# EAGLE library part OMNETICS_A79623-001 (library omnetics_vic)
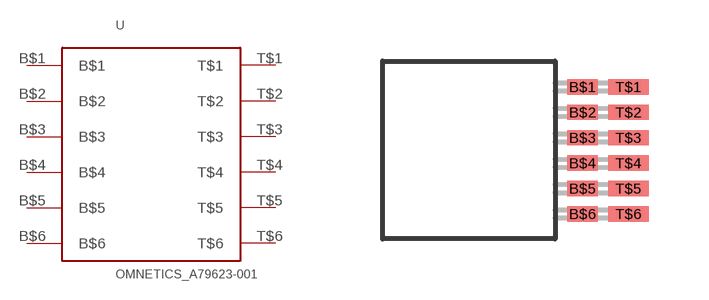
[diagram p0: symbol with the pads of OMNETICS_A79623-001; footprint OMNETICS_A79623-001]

Designator prefix -

## OMNETICS_A79623-001  [OMNETICS_A79623-001]
B$1  B$1
B$2  B$2
B$3  B$3
B$4  B$4
B$5  B$5
B$6  B$6
T$1  T$1
T$2  T$2
T$3  T$3
T$4  T$4
T$5  T$5
T$6  T$6

## Footprint OMNETICS_A79623-001 (pad centres in mm)
Omnetics PZN-12-AA 12 pin footprint
smd 0.762 x 0.381: B$1 2.845,1.575; B$2 2.845,0.94; B$3 2.845,0.305; B$4 2.845,-0.33; B$5 2.845,-0.965; B$6 2.845,-1.6
smd 1.016 x 0.381: T$1 3.988,1.575; T$2 3.988,0.94; T$3 3.988,0.305; T$4 3.988,-0.33; T$5 3.988,-0.965; T$6 3.988,-1.6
